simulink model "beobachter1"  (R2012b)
settings: Solver=ode45  StartTime=0.0  StopTime=10.0  RelTol=1e-3
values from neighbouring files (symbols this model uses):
  A = [0 1 0 0 0 0    [beobachter_1.m]    (also in beobachter_2.m; beobachter_22.m; kalman_1.m = my_sys.a; kalman_10.m = my_sys.a)
  B = [0 1 0 0 0 0]'    [beobachter_1.m]    (also in beobachter_2.m; beobachter_22.m; kalman_1.m = my_sys.b; kalman_10.m = my_sys.b)
  C = [0 0 0 0 1 0]    [beobachter_1.m]    (also in beobachter_2.m; beobachter_22.m; kalman_1.m = my_sys.c; kalman_10.m = my_sys.c)
  D = 0    [aktiv_tilger_1.m]    (also in aktiv_tilger_12.m; aktiv_tilger_3.m = 2000; aktiv_tilger_31.m; beobachter_1.m)
  Ke = (place(A',C',p))'    [beobachter_1.m]    (also in beobachter_2.m; beobachter_22.m)
  x0 = [30,-20,0,0,0,0]    [beobachter_1.m]    (also in beobachter_2.m = [0,0,0,0,0.3,0]; beobachter_22.m = [0.1,0,0.1,0,0.3,0]; kalman_13.m = zeros(1,3); kalman_d1.m = zeros(1,3))

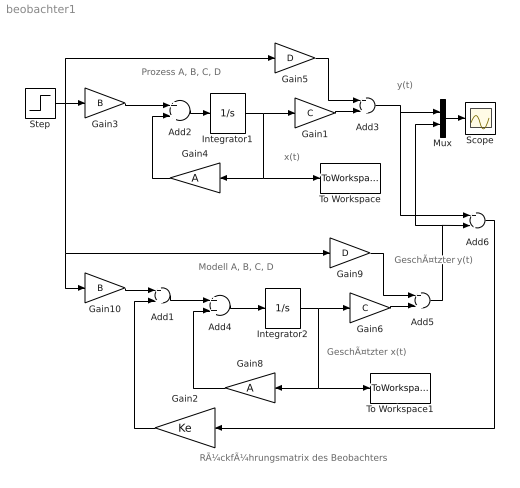
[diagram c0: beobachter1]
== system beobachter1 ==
  note: GeschÃ¤tzter
  note: y(t)
  note: x(t)
  note: Prozess A, B, C, D
  note: y(t)
  note: GeschÃ¤tzter x(t)
  note: RÃ¼ckfÃ¼hrungsmatrix des Beobachters
  note: Modell A, B, C, D
  Add{1..5} (5 alike) : Sum
  Add6 : Sum  Inputs=+-
  Gain1 : Gain  Gain=C  Multiplication=Matrix(K*u)
  Gain10 : Gain  Gain=B  Multiplication=Matrix(K*u)
  Gain2 : Gain  Gain=Ke  Multiplication=Matrix(K*u)
  Gain3 : Gain  Gain=B  Multiplication=Matrix(K*u)
  Gain4 : Gain  Gain=A  Multiplication=Matrix(K*u)
  Gain5 : Gain  Gain=D  Multiplication=Matrix(K*u)
  Gain6 : Gain  Gain=C  Multiplication=Matrix(K*u)
  Gain8 : Gain  Gain=A  Multiplication=Matrix(K*u)
  Gain9 : Gain  Gain=D  Multiplication=Matrix(K*u)
  Integrator1 : Integrator  InitialCondition=x0
  Integrator2 : Integrator
  Mux : Mux  Inputs=2
  Scope : Scope
  Step : Step  SampleTime=0
  To Workspace : ToWorkspace  VariableName=x  SampleTime=-1  SaveFormat=Structure With Time
  To Workspace1 : ToWorkspace  VariableName=x1  SampleTime=-1  SaveFormat=Structure With Time
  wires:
  Integrator1/1 -> Gain1/1, To Workspace/1, Gain4/1
  Gain1/1 -> Add3/2
  Add2/1 -> Integrator1/1
  Gain3/1 -> Add2/1
  Gain4/1 -> Add2/2
  Add3/1 -> Mux/1, Add6/1
  Step/1 -> Gain3/1, Gain10/1, Gain9/1, Gain5/1
  Gain5/1 -> Add3/1
  Integrator2/1 -> Gain8/1, To Workspace1/1, Gain6/1
  Gain2/1 -> Add1/2
  Gain6/1 -> Add5/2
  Add4/1 -> Integrator2/1
  Add1/1 -> Add4/1
  Gain8/1 -> Add4/2
  Gain9/1 -> Add5/1
  Gain10/1 -> Add1/1
  Add6/1 -> Gain2/1
  Mux/1 -> Scope/1
  Add5/1 -> Mux/2, Add6/2
